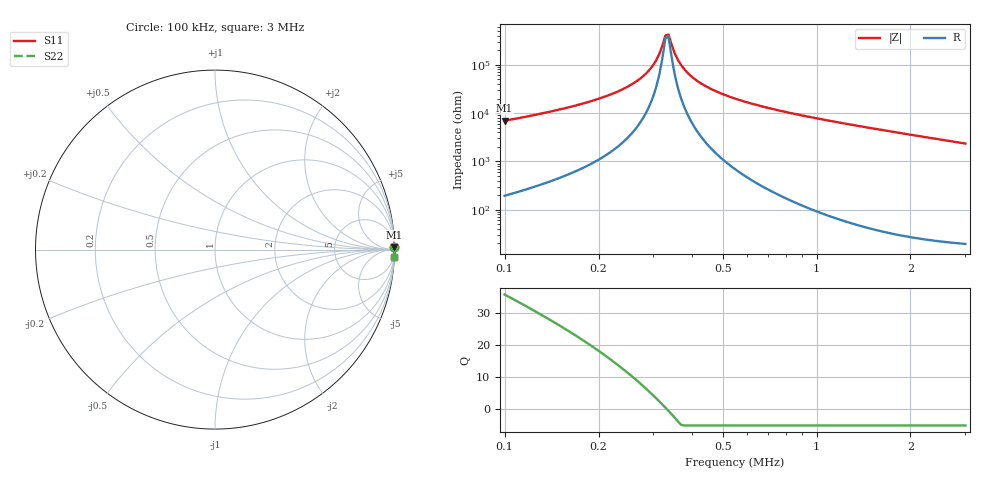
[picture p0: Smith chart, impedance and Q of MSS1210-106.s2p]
# MHz S MA R 50
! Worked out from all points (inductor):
!   150 points, 100 kHz to 3 MHz, reference 50 ohm
!   read as one part in series: L = 9.96 mH near 100 kHz
!   highest Q = 35.7 at 100 kHz (marker M1), where L = 11 mH
!   self-resonance near 327.7 kHz
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0.1  0.9995 0.8  0.01447 -87.6  0.01447 -87.6  0.9995 0.8
0.2173008  0.9997 0.2  0.004191 -86.1  0.004191 -86.1  0.9997 0.2
0.2668599  0.9998 0.1  0.002121 -83.4  0.002121 -83.4  0.9998 0.1
0.2857749  0.9998 0.1  0.001458 -80.8  0.001458 -80.8  0.9998 0.1
0.2991239  0.9998 0.1  0.001023 -77.2  0.001023 -77.2  0.9998 0.1
0.3130965  0.9998 0.0  0.0006009 -68.3  0.0006009 -68.3  0.9998 0.0
0.3277219  0.9998 0.0  0.0002479 -29.1  0.0002479 -29.1  0.9998 0.0
0.3352887  0.9998 -0.0  0.0002358 24.7  0.0002358 24.7  0.9998 -0.0
0.3509507  0.9998 -0.0  0.000576 68.6  0.000576 68.6  0.9998 -0.0
0.3590539  0.9998 -0.0  0.0007839 74.6  0.0007839 74.6  0.9998 -0.0
0.375826  0.9998 -0.1  0.001213 80.3  0.001213 80.3  0.9998 -0.1
0.4024644  0.9998 -0.1  0.001871 83.9  0.001871 83.9  0.9998 -0.1
0.430991  0.9998 -0.1  0.002542 85.5  0.002542 85.5  0.9998 -0.1
0.4721962  0.9998 -0.2  0.003457 86.8  0.003457 86.8  0.9998 -0.2
0.5292858  0.9998 -0.3  0.004644 87.6  0.004644 87.6  0.9998 -0.3
0.5932778  0.9998 -0.3  0.005892 88.0  0.005892 88.0  0.9998 -0.3
0.7982418  0.9998 -0.5  0.009541 88.5  0.009541 88.5  0.9998 -0.5
1.074016  0.9997 -0.8  0.01404 88.6  0.01404 88.6  0.9997 -0.8
1.583221  0.9996 -1.3  0.02187 88.3  0.02187 88.3  0.9996 -1.3
2.035123  0.9994 -1.6  0.02861 87.9  0.02861 87.9  0.9994 -1.6
2.556974  0.9991 -2.1  0.03629 87.5  0.03629 87.5  0.9991 -2.1
3  0.9987 -2.5  0.04277 87.1  0.04277 87.1  0.9987 -2.5
